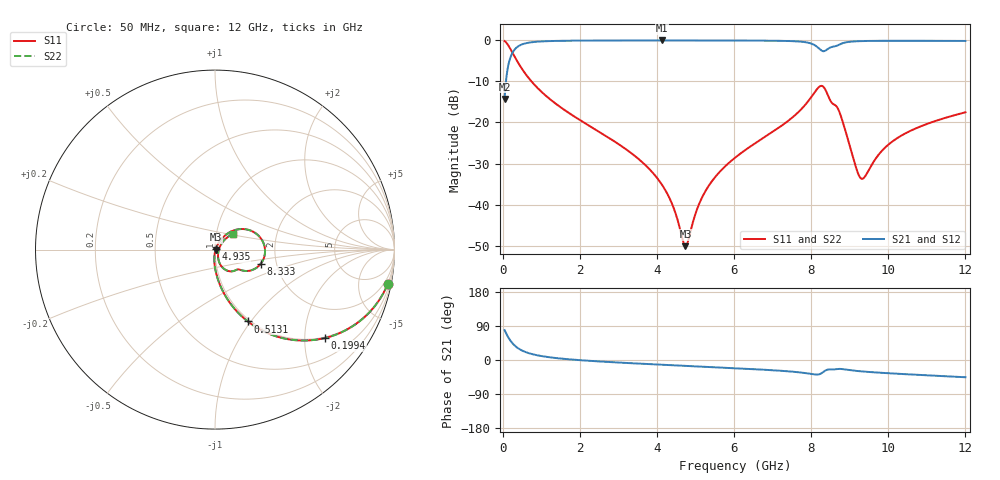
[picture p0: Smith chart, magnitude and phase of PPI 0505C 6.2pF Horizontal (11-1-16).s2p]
# MHz S MA R 50
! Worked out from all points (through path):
!   1601 points, 50 MHz to 12 GHz, reference 50 ohm
!   highest |S21| = -0.03 dB at 4.12 GHz (marker M1); lowest = -14.3 dB at 50 MHz (marker M2)
!   group delay of S21, straight-line fit = 14.8 ps
!   lowest |S11| = -50.1 dB at 4.74 GHz (marker M3), VSWR 1.01, Z = 50.3 - j0.0958 ohm
!   |S11| at or under -10 dB: 746.8 MHz to end of sweep
!   |S22| runs from -50.1 to -0.2 dB; largest |S21 - S12| = 0
!   S11 on the Smith chart (normalised r, x): 50 MHz: 1, -10; 199.4 MHz: 0.97, -2.51; 513.1 MHz: 0.97, -0.97; 4.935 GHz: 1.01, +0.01; 8.333 GHz: 1.65, -0.28; 12 GHz: 1.20, +0.21
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50  0.9812 -11.3  0.1928 78.7  0.1928 78.7  0.9812 -11.3
199.375  0.7864 -38.8  0.6171 51.2  0.6171 51.2  0.7864 -38.8
341.2812  0.5957 -54.5  0.8024 35.4  0.8024 35.4  0.5957 -54.5
513.0625  0.4405 -65.4  0.8967 24.5  0.8967 24.5  0.4405 -65.4
991.0625  0.2399 -79.0  0.9693 10.6  0.9693 10.6  0.2399 -79.0
2044.156  0.1042 -89.6  0.9925 -0.7  0.9925 -0.7  0.1042 -89.6
3343.719  0.04202 -95.1  0.9964 -8.5  0.9964 -8.5  0.04202 -95.1
4038.312  0.02012 -94.1  0.9968 -12.0  0.9968 -12.0  0.02012 -94.1
4120.469  0.01776 -93.3  0.9968 -12.4  0.9968 -12.4  0.01776 -93.3
4404.281  0.009898 -86.5  0.9967 -13.8  0.9967 -13.8  0.009898 -86.5
4740.375  0.00312 -17.8  0.9966 -15.4  0.9966 -15.4  0.00312 -17.8
4934.562  0.006134 41.9  0.9964 -16.4  0.9964 -16.4  0.006134 41.9
5337.875  0.0168 59.7  0.996 -18.3  0.996 -18.3  0.0168 59.7
6025  0.03721 61.8  0.9947 -21.7  0.9947 -21.7  0.03721 61.8
7451.531  0.109 52.7  0.9802 -30.2  0.9802 -30.2  0.109 52.7
8019.156  0.209 32.5  0.9074 -37.1  0.9074 -37.1  0.209 32.5
8332.844  0.2667 -17.3  0.7377 -30.2  0.7377 -30.2  0.2667 -17.3
8728.688  0.1358 -59.8  0.887 -23.4  0.887 -23.4  0.1358 -59.8
9288.844  0.02089 -22.2  0.9787 -29.9  0.9787 -29.9  0.02089 -22.2
10013.31  0.05424 43.8  0.9874 -35.0  0.9874 -35.0  0.05424 43.8
10782.59  0.08744 45.4  0.9874 -39.2  0.9874 -39.2  0.08744 45.4
12000  0.1331 41.4  0.9831 -45.5  0.9831 -45.5  0.1331 41.4
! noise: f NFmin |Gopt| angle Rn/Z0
50  0.0005387  0.9065  1.669  0.001265
1372  0.004806  0.7223  5.028  0.003425
2701  0.007861  0.6754  9.143  0.004642
4031  0.01071  0.651  13.26  0.005755
5360  0.01388  0.6453  17.32  0.007251
6682  0.01969  0.6835  21.36  0.01166
8012  0.07694  0.8918  25.7  0.1472
9341  0.04182  0.7833  29.86  0.03704
1.067e+04  0.02963  0.6755  33.53  0.0162
1.2e+04  0.02935  0.6432  37.09  0.01406
